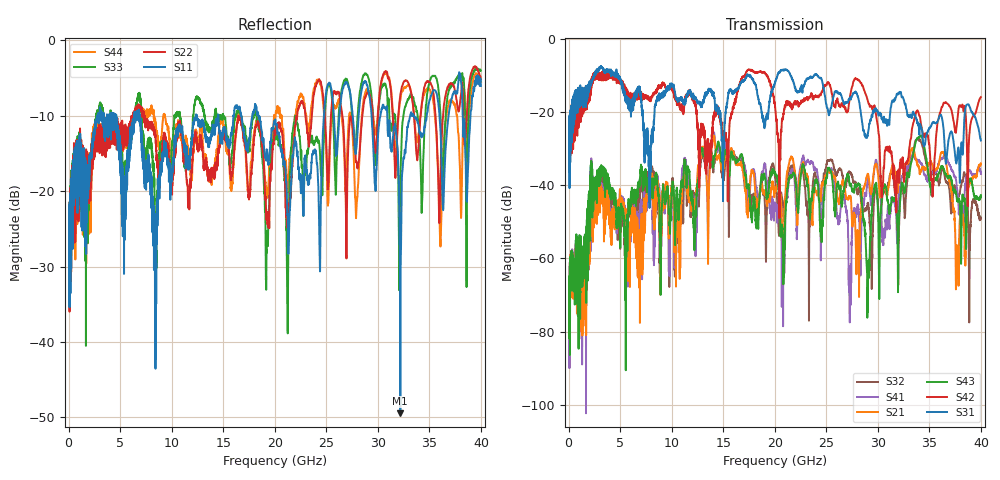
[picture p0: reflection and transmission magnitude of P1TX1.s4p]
!Agilent Technologies,N5245A,MY49151084,A.09.20.08
!Agilent N5245A: A.09.20.08
!Date: Thursday, March 01, 2012 13:57:32
!Correction: S11(Full 4 Port(1,2,3,4))
!S12(Full 4 Port(1,2,3,4))
!S13(Full 4 Port(1,2,3,4))
!S14(Full 4 Port(1,2,3,4))
!S21(Full 4 Port(1,2,3,4))
!S22(Full 4 Port(1,2,3,4))
!S23(Full 4 Port(1,2,3,4))
!S24(Full 4 Port(1,2,3,4))
!S31(Full 4 Port(1,2,3,4))
!S32(Full 4 Port(1,2,3,4))
!S33(Full 4 Port(1,2,3,4))
!S34(Full 4 Port(1,2,3,4))
!S41(Full 4 Port(1,2,3,4))
!S42(Full 4 Port(1,2,3,4))
!S43(Full 4 Port(1,2,3,4))
!S44(Full 4 Port(1,2,3,4))
!S4P File: Measurements: <S11,S12,S13,S14>,
!<S21,S22,S23,S24>,
!<S31,S32,S33,S34>,
!<S41,S42,S43,S44>:
# Hz S  dB  R 50
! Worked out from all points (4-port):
!   3996 points, 50 MHz to 40 GHz, reference 50 ohm
!   strongest paths, dB at 50 MHz, 10.04 GHz, 20.03 GHz, 30.02 GHz, 40 GHz:
!     S31: -23.7, -12.9, -12.0, -20.3, -27.7
!     S42: -24.7, -13.8, -18.6, -24.2, -15.9
!     S43: -65.0, -41.4, -36.5, -47.5, -42.7
!     S21: -76.9, -40.9, -41.6, -36.7, -34.0
!     S41: -68.8, -43.3, -45.8, -36.0, -36.9
!     S32: -71.5, -39.4, -37.7, -45.6, -48.9
!   lowest |S11| = -49.5 dB at 32.18 GHz (marker M1), VSWR 1.01, Z = 50.2 - j0.26 ohm
!   |S11| at or under -10 dB: start of sweep to 2.819 GHz; 6.92 GHz to 12.34 GHz (5.423 GHz wide, 56.3 % of centre); 18.42 GHz to 24.76 GHz (6.342 GHz wide, 29.4 % of centre)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
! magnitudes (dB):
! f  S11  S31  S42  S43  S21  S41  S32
! 50 MHz  -23.7  -23.7  -24.7  -65.0  -76.9  -68.8  -71.5
! 3.22 GHz  -9.7  -7.8  -10.9  -36.4  -44.1  -41.5  -38.3
! 23.53 GHz  -17.1  -10.4  -15.0  -43.7  -46.2  -33.4  -45.7
! 27.31 GHz  -7.0  -16.0  -15.6  -39.9  -43.3  -62.1  -36.5
! 32.18 GHz  -49.5  -14.5  -33.5  -44.1  -35.0  -40.3  -42.9
! 37.71 GHz  -7.0  -32.4  -22.3  -44.1  -56.7  -41.0  -42.5
! 40 GHz  -6.1  -27.7  -15.9  -42.7  -34.0  -36.9  -48.9
